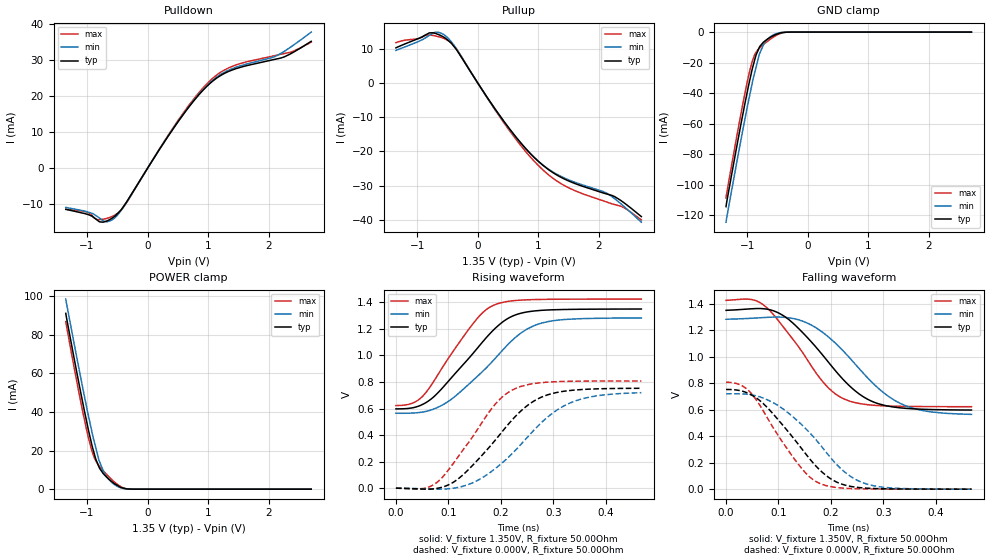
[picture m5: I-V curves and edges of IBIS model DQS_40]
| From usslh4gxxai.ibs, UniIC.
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| MODEL DQS_40 (40 Ohm Data Strobe I/O with no ODT, 800-2133Mbps)
[Model]   DQS_40
Model_type   I/O
Vinl = 545.000mV
Vinh = 805.000mV
Vmeas = 675.000mV
Vref = 675.000mV
Cref = 0.0pF
Rref = 25.000Ohm
|   typ   min   max
|C_comp   1.050pF   1.000pF   1.100pF
C_comp_pullup   0.5250pF   0.5000pF   0.5500pF
C_comp_pulldown   0.5250pF   0.5000pF   0.5500pF
[Model Spec]
| Input threshold voltage corners
Vinl   0.5450V   0.5115V   0.5825V
Vinh   0.8050V   0.7715V   0.8425V
| Measurement voltage corners
Vmeas   0.6750V   0.6415V   0.7125V
| Timing spec test load voltage corners
Vref   0.6750V   0.6415V   0.7125V
| Dynamic Overshoot Parameters from DDR3L Specification
|D_overshoot_ampl_h   0.40   NA   NA
|D_overshoot_ampl_l   0.40   NA   NA
|D_overshoot_area_h   0.11n   NA   NA
|D_overshoot_area_l   0.11n   NA   NA
[Receiver Thresholds]
|Vth   =  0.675V
|Vth_min  =  0.6615V
|Vth_max  =  0.6885V
|Vinh_ac  =  0.130V
|Vinh_dc  =  0.090V
|Vinl_ac  = -0.130V
|Vinl_dc  = -0.090V
|Tslew_ac =  5.000ns |Not specified, so set to high value
|Threshold_sensitivity = 0.50
|Reference_supply Pullup_ref
|NOTE: If using the IBISCHK 4.2.1 or older parser, Differential receiver
|threshold parameters must be commented out because the parser generates
|errors for multiple differential models.
Vcross_low   = 0.545V
Vcross_high  = 0.805V
Vdiff_ac   = 260mV
Vdiff_dc   = 180mV
Tdiffslew_ac = 10.000ns |Not specified, so set to high value
[Voltage Range]   1.3500V   1.2830V   1.4250V
[Pullup Reference]   1.3500V   1.2830V   1.4250V
[Temperature Range]   45.0   95.0   -40.0
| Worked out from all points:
|   slope of the pulldown table from 0 to 0.203 V, typ, clamps not added: 37.7 ohm
|   slope of the pullup table from 0 to 0.203 V, typ, clamps not added: 37.4 ohm
|   GND clamp passes 1 mA (typ) near -0.48 V on its own axis
|   POWER clamp passes 1 mA (typ) near -0.45 V on its own axis
|   falling waveform, V_fixture 1.350V, R_fixture 50.00Ohm: 20-80 % time 103ps typ, 109ps min, 89.3ps max; typ from 1.35 V to 0.597 V
|   rising waveform, V_fixture 1.350V, R_fixture 50.00Ohm: 20-80 % time 101ps typ, 111ps min, 83.6ps max; typ from 0.597 V to 1.35 V
|   rising waveform, V_fixture 0.000V, R_fixture 50.00Ohm: 20-80 % time 103ps typ, 114ps min, 87.6ps max; typ from 0 V to 0.753 V
|   falling waveform, V_fixture 0.000V, R_fixture 50.00Ohm: 20-80 % time 95.3ps typ, 103ps min, 80.9ps max; typ from 0.753 V to 0 V
[Pulldown]
|   Voltage   I(typ)   I(min)   I(max)
-1.35V    -11.4mA    -10.87mA   -11.42mA
-1.015V   -12.69mA   -12mA      -12.09mA
-795mV    -14.86mA   -13.8mA    -14.27mA
-665mV    -14.56mA   -14.83mA   -13.86mA
-560mV    -13.55mA   -14.01mA   -13.18mA
-385mV    -10.3mA    -10.43mA   -10.51mA
515mV     13.14mA    13.2mA     13.49mA
1.05V     23.74mA    23.97mA    24.5mA
1.445V    27.45mA    27.84mA    28.48mA
2.13V     30.22mA    31.11mA    31.26mA
2.365V    31.7mA     33.56mA    32.12mA
2.7V      35.1mA     37.65mA    34.88mA
[GND Clamp]
|   Voltage   I(typ)   I(min)   I(max)
-1.35V    -114.4mA   -124.6mA   -108.7mA
-1.245V   -90.61mA   -100.9mA   -84.29mA
-1.105V   -60.48mA   -70.85mA   -53.72mA
-1.015V   -42.18mA   -52.23mA   -35.44mA
-925mV    -25.46mA   -34.83mA   -20.16mA
-875mV    -17.89mA   -26.12mA   -14.58mA
-800mV    -9.934mA   -14.48mA   -10.56mA
-715mV    -6.057mA   -6.91mA    -7.57mA
-615mV    -3.335mA   -2.939mA   -4.509mA
-490mV    -1.072mA   -664.8uA   -1.477mA
-345mV    -47.71uA   -29.49uA   -74.91uA
2.7V      0A         0A         0A
[Pullup]
|   Voltage   I(typ)   I(min)   I(max)
-1.35V    10.26mA    9.507mA    11.78mA
-795mV    14.65mA    13.96mA    14.01mA
-665mV    14.28mA    14.87mA    13.61mA
-560mV    13.37mA    14.13mA    13.04mA
-350mV    9.722mA    9.924mA    9.925mA
535mV     -13.63mA   -13.74mA   -14.18mA
810mV     -19.51mA   -19.57mA   -20.42mA
1.085V    -24.19mA   -24.11mA   -25.56mA
1.495V    -28.59mA   -28.27mA   -30.59mA
2.13V     -32.45mA   -32.23mA   -34.81mA
2.42V     -35.1mA    -36.18mA   -36.52mA
2.7V      -39.05mA   -40.69mA   -40.03mA
[POWER Clamp]
|   Voltage   I(typ)   I(min)   I(max)
-1.35V    91.15mA    98.58mA    86.92mA
-1.245V   73.24mA    80.85mA    68.58mA
-1.105V   50.34mA    58.03mA    45.63mA
-1.015V   36.4mA     43.87mA    32.02mA
-920mV    22.95mA    29.85mA    19.9mA
-855mV    15.55mA    21.44mA    14.76mA
-800mV    11.29mA    14.78mA    12.09mA
-720mV    7.69mA     8.611mA    9.138mA
-560mV    3.172mA    2.652mA    4.06mA
-430mV    798.9uA    593.6uA    1.064mA
-305mV    80.62uA    46.1uA     58.38uA
2.7V      0A         0A         0A
[Ramp]
R_load = 50.00Ohm
|   typ   min   max
dV/dt_r   451.595mV/103.216ps 431.697mV/114.150ps 484.432mV/87.545ps
dV/dt_f   451.543mV/102.727ps 431.065mV/108.923ps 481.359mV/89.346ps
[Falling Waveform]
V_fixture = 1.350V
V_fixture_min = 1.283V
V_fixture_max = 1.425V
R_fixture = 50.00Ohm
|   Time   V(typ)   V(min)   V(max)
0s        1.35V      1.283V     1.425V
60ps      1.364V     1.293V     1.418V
108ps     1.313V     1.298V     1.231V
166ps     1.097V     1.231V     910.2mV
196ps     954.9mV    1.147V     761.3mV
226ps     816.9mV    1.033V     679.2mV
276ps     666.9mV    815.7mV    635.4mV
334ps     613.2mV    644.3mV    625.3mV
382ps     602.2mV    588.7mV    623.4mV
468ps     597.4mV    564.6mV    622.7mV
[Rising Waveform]
V_fixture = 1.350V
V_fixture_min = 1.283V
V_fixture_max = 1.425V
R_fixture = 50.00Ohm
|   Time   V(typ)   V(min)   V(max)
0s        597.4mV    564.6mV    622.7mV
38ps      611.5mV    567.6mV    652.9mV
68ps      674.6mV    590.4mV    780.2mV
102ps     814.8mV    659.6mV    990.4mV
146ps     1.011V     809mV      1.234V
186ps     1.192V     963.7mV    1.378V
226ps     1.303V     1.129V     1.413V
276ps     1.34V      1.242V     1.422V
324ps     1.347V     1.272V     1.424V
468ps     1.35V      1.283V     1.425V
[Rising Waveform]
V_fixture = 0.000V
V_fixture_min = 0.000V
V_fixture_max = 0.000V
R_fixture = 50.00Ohm
|   Time   V(typ)   V(min)   V(max)
0s        -2.121uV   -29.43uV   -13.18uV
66ps      -6.977mV   -6.127mV   14.04mV
108ps     41.2mV     -1.192mV   178.9mV
148ps     179.2mV    43.53mV    397.1mV
188ps     355mV      143.3mV    626.4mV
228ps     541.5mV    286.2mV    751.1mV
276ps     683.3mV    488.5mV    794.6mV
332ps     736.1mV    641.8mV    805.3mV
382ps     748.2mV    695.1mV    807.2mV
468ps     752.7mV    719.5mV    807.5mV
[Falling Waveform]
V_fixture = 0.000V
V_fixture_min = 0.000V
V_fixture_max = 0.000V
R_fixture = 50.00Ohm
|   Time   V(typ)   V(min)   V(max)
0s        752.7mV    719.5mV    807.5mV
36ps      733.6mV    718.1mV    767mV
68ps      656.5mV    691.9mV    610.4mV
100ps     521.1mV    629.2mV    401.2mV
136ps     347.8mV    516.6mV    197.8mV
158ps     236.2mV    432.4mV    97.63mV
178ps     147.7mV    342.5mV    44.69mV
226ps     31.55mV    130.2mV    7.017mV
272ps     6.684mV    34.56mV    1.736mV
468ps     -2.121uV   -29.43uV   -13.18uV
